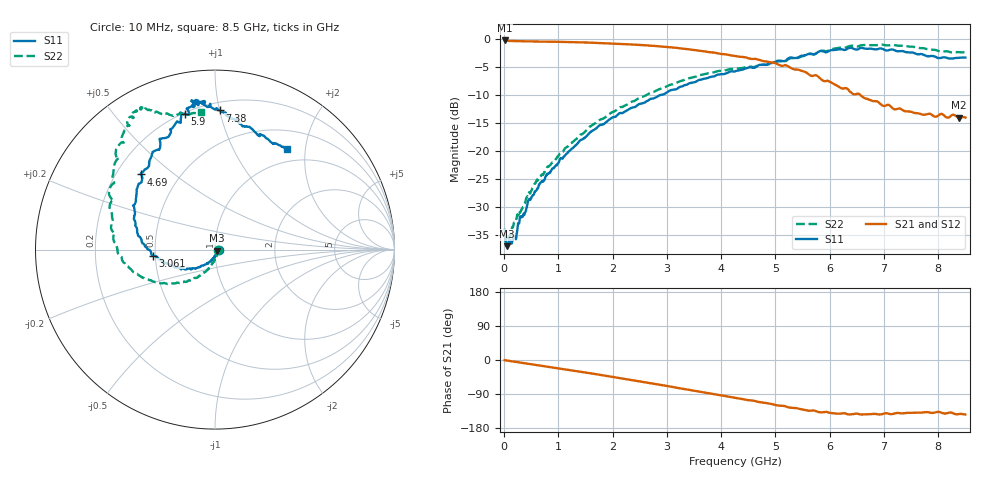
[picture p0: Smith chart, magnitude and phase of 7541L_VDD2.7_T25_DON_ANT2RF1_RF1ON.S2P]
!Agilent Technologies,E5071C,MY46417908,A.11.23
!Date: Wed Dec 09 17:17:10 2020
!Data & Calibration Information:
!Freq	S11:SOLT2(ON)	S21:SOLT2(ON)	S12:SOLT2(ON)	S22:SOLT2(ON)
!PortZ  Port1:50+j0  Port2:50+j0
!Above PortZ is port z conversion or system Z0 setting when saving the data.
!When reading, reference impedance value at option line is always used.
# Hz S dB R 50
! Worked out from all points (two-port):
!   1601 points, 10 MHz to 8.5 GHz, reference 50 ohm
!   highest |S21| = -0.19 dB at 10 MHz (marker M1); lowest = -14.1 dB at 8.383 GHz (marker M2)
!   |S21| within 3 dB of the highest: start of sweep to 4.434 GHz
!   lowest |S11| = -37.1 dB at 47.14 MHz (marker M3), VSWR 1.03, Z = 51.3 - j0.589 ohm
!   |S11| at or under -10 dB: start of sweep to 2.87 GHz
!   |S22| runs from -36.2 to -0.9 dB; largest |S21 - S12| = 0.0036
!   S11 on the Smith chart (normalised r, x): 10 MHz: 1.04, -0.00; 3.061 GHz: 0.48, -0.04; 4.69 GHz: 0.30, +0.39; 5.9 GHz: 0.21, +0.78; 7.38 GHz: 0.26, +1.00; 8.5 GHz: 0.79, +1.67
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1e7  -34.17 -2.9  -0.19 -0.5  -0.19 -0.5  -35.46 -12.5
4.714375e7  -37.09 -24.3  -0.26 -1.3  -0.26 -1.3  -35.93 -25.7
1.851062e8  -35.45 -59.9  -0.30 -4.3  -0.31 -4.3  -32.92 -54.5
2.912312e8  -31.95 -75.3  -0.32 -6.6  -0.32 -6.7  -31.13 -71.4
5.777688e8  -27.25 -96.0  -0.38 -12.7  -0.38 -12.7  -25.81 -89.2
1.050025e9  -21.29 -115.9  -0.45 -23.0  -0.46 -23.0  -20.23 -105.2
1.426769e9  -17.99 -129.8  -0.54 -31.4  -0.54 -31.4  -17.05 -116.2
2.111275e9  -13.31 -150.3  -0.80 -47.0  -0.80 -47.0  -12.35 -131.9
2.843538e9  -10.13 -169.7  -1.24 -64.7  -1.24 -64.7  -9.01 -148.1
3.061094e9  -9.14 -174.5  -1.42 -70.0  -1.42 -70.0  -8.12 -153.6
3.644781e9  -7.18 168.9  -2.09 -84.7  -2.08 -84.7  -6.36 -166.8
4.255e9  -5.73 148.6  -2.97 -99.7  -2.96 -99.7  -5.29 179.6
4.690112e9  -4.63 134.5  -3.65 -110.7  -3.66 -110.7  -4.60 168.8
5.236656e9  -3.40 116.9  -4.84 -124.9  -4.83 -124.9  -3.56 152.6
5.671769e9  -2.64 106.0  -6.57 -133.2  -6.52 -133.2  -2.61 136.8
5.899938e9  -2.23 102.4  -7.49 -137.4  -7.44 -137.1  -2.06 130.8
6.414644e9  -1.57 98.9  -9.69 -143.1  -9.71 -142.8  -1.13 122.6
7.088538e9  -1.92 92.2  -11.74 -141.9  -11.78 -142.1  -1.06 118.0
7.380381e9  -2.21 88.1  -12.86 -140.4  -12.86 -140.2  -1.16 116.1
7.884475e9  -2.99 74.8  -13.55 -139.8  -13.58 -139.7  -1.88 111.0
8.383262e9  -3.30 56.9  -14.06 -142.5  -14.08 -142.7  -2.28 98.7
8.5e9  -3.26 54.3  -14.02 -143.9  -14.10 -143.9  -2.28 95.7
